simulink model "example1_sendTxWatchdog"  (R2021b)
settings: Solver=FixedStepDiscrete  StartTime=0.0  StopTime=inf  FixedStep=0.5  RelTol=1e-3
libraries: CANBusLib x3

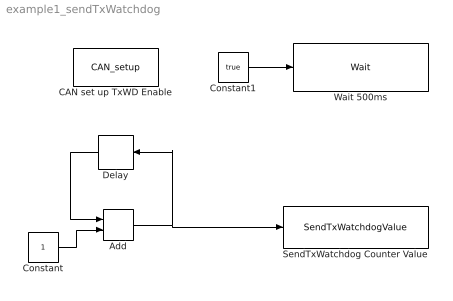
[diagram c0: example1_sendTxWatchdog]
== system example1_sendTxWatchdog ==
  Add : Sum
  CAN set up TxWD Enable : CANBusLib/CAN_setup  Priority=1  g1_cmbPortName="\"COM17\""  g2_cmbBaudRate=250000  g3_chkEcho=off  g59_chkTerminator=on  g4_cmbObjectID=0  g5_chkEnableSync=off  g10_chkRxWDEnable=off  g12_cmbRxWDLen=1  g13_cmbRxWDStartPos=1  g_60_cmbRxWDMode=0  g15_chkTxWDEnable=on  g17_cmbTxWDLen=1  g18_cmbTxWDStartPos=1  g_61_cmbTxWDMode=0  g20_ediF1=0  g21_chkExt4F1=off  g22_ediF2=0  g23_chkExt4F2=off  g24_ediF3=0  g25_chkExt4F3=off  g26_ediF4=0  g27_chkExt4F4=off  g28_ediF5=0  g29_chkExt4F5=off  g30_ediF6=0  g31_chkExt4F6=off  g32_ediF7=0  g33_chkExt4F7=off  g34_ediF8=0  g35_chkExt4F8=off  g36_ediM1=0  g37_ediF9=0  g38_chkExt4F9=on  g39_ediF10=0  g40_chkExt4F10=on  g41_ediF11=0  g42_chkExt4F11=on  g43_ediF12=0  g44_chkExt4F12=on  g45_ediM2=0  g46_ediF13=0  g47_chkExt4F13=off  g48_ediF14=0  g49_chkExt4F14=on  g50_ediF15=0  g51_chkExt4F15=on  g52_ediF16=0  g53_chkExt4F16=on  g54_ediM3=0  g62_autoFresh=on
  Constant : Constant
  Constant1 : Constant  Value=true
  Delay : Delay  DelayLength=1
  SendTxWatchdog Counter Value : CANBusLib/SendTxWatchdogValue  g1_cmbObjectID=0
  Wait 500ms : CANBusLib/Wait  Waitms=500
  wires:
  Add/1 -> Delay/1, SendTxWatchdog Counter Value/1
  Delay/1 -> Add/1
  Constant/1 -> Add/2
  Constant1/1 -> Wait 500ms/1
